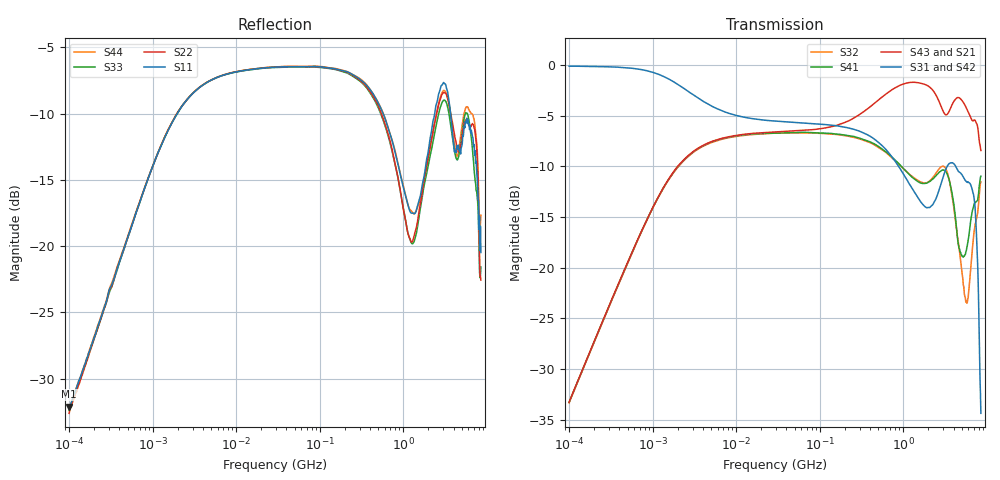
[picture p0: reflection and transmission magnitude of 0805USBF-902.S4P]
# Hz S dB R 50
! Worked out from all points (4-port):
!   801 points, 100 kHz to 8.5 GHz, reference 50 ohm
!   strongest paths, dB at 100 kHz, 1.721 MHz, 29.51 MHz, 502.3 MHz, 8.5 GHz:
!     S31: -0.1, -1.6, -5.5, -7.6, -34.4
!     S42: -0.1, -1.5, -5.5, -7.6, -32.7
!     S43: -33.3, -10.7, -6.6, -3.4, -8.4
!     S21: -33.3, -10.7, -6.6, -3.5, -8.8
!     S41: -33.3, -10.7, -6.7, -8.0, -11.0
!     S32: -33.3, -10.8, -6.7, -8.1, -11.5
!   lowest |S11| = -32.1 dB at 100 kHz (marker M1), VSWR 1.05, Z = 50.7 + j2.4 ohm
!   |S11| at or under -10 dB: start of sweep to 1.969 MHz; 574.9 MHz to 2.379 GHz (1.804 GHz wide, 122 % of centre); 3.679 GHz to end of sweep
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100000  -32.10 72.0  -33.26 86.8  -0.09 -1.3  -33.31 -93.2
        -33.28 86.8  -32.61 70.9  -33.35 -93.1  -0.07 -1.2
        -0.09 -1.3  -33.34 -93.3  -32.40 66.4  -33.31 86.8
        -33.31 -93.4  -0.07 -1.2  -33.28 86.8  -32.27 72.6
2.856676e8  -7.29 -61.0  -5.00 -31.7  -6.45 -75.4  -7.15 104.2
            -5.01 -31.7  -7.37 -63.1  -7.22 102.4  -6.46 -75.2
            -6.45 -75.4  -7.22 102.3  -7.43 -63.3  -4.99 -31.6
            -7.14 104.2  -6.45 -75.2  -4.98 -31.6  -7.26 -61.3
1.127919e9  -16.82 168.5  -1.73 178.6  -11.43 91.1  -10.62 -92.3
            -1.73 178.6  -18.95 166.4  -10.59 -96.8  -11.38 90.4
            -11.44 91.1  -10.60 -96.8  -18.90 167.3  -1.74 178.4
            -10.62 -92.2  -11.38 90.4  -1.73 178.4  -16.79 167.2
2.04983e9  -12.26 58.9  -2.17 12.1  -14.05 -106.4  -11.49 82.5
           -2.17 12.1  -12.84 63.4  -11.45 76.9  -14.13 -105.3
           -14.05 -106.4  -11.45 76.9  -13.51 59.6  -2.13 12.9
           -11.50 82.5  -14.13 -105.5  -2.13 12.9  -12.95 56.4
3.154505e9  -7.75 -148.5  -5.30 -169.7  -10.51 -3.3  -10.40 -157.7
            -5.30 -169.8  -8.44 -151.0  -10.07 -162.8  -10.49 -1.7
            -10.50 -3.3  -10.08 -162.8  -9.01 -152.0  -4.83 -169.8
            -10.40 -157.8  -10.47 -1.7  -4.83 -169.7  -8.30 -146.5
4.263844e9  -12.96 23.0  -3.78 14.4  -10.00 103.8  -15.44 -63.3
            -3.78 14.3  -12.07 9.7  -15.73 -51.6  -10.48 107.2
            -10.02 103.8  -15.74 -51.5  -13.32 19.3  -3.32 11.8
            -15.44 -63.3  -10.47 107.3  -3.31 11.9  -12.95 22.7
8.5e9  -20.48 25.5  -8.76 10.4  -35.27 -5.7  -11.01 84.5
       -8.78 10.5  -22.57 33.9  -11.53 76.9  -32.04 -62.2
       -34.38 -8.5  -11.52 77.3  -21.58 9.2  -8.43 2.5
       -10.96 84.6  -32.66 -62.2  -8.42 1.9  -17.67 29.8
